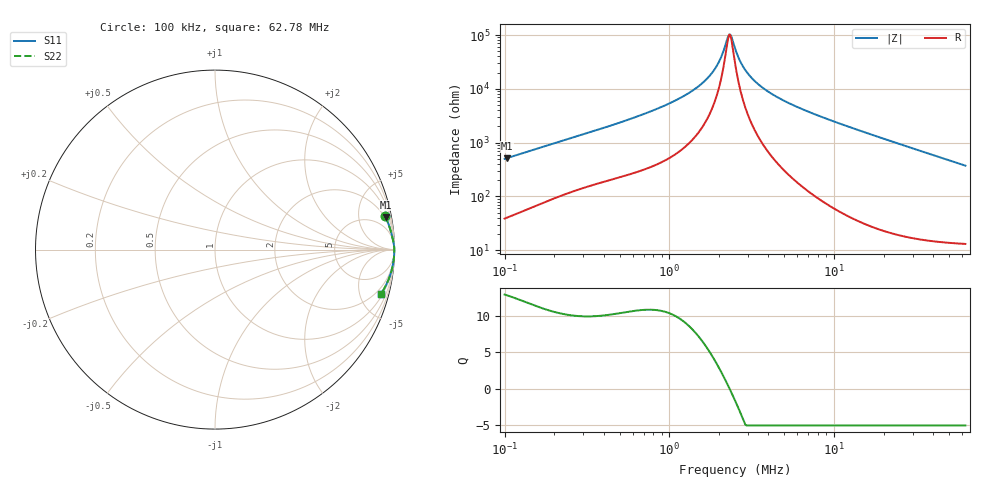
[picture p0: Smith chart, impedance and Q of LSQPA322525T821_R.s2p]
! LSQPA322525T821_R  S-PARAMETER MODEL  ( General Type )
! Model Generated by TAIYO YUDEN Corporation (http://www.ty-top.com)
! Version 1.0
! TAIYO YUDEN Control No. 111018NG25SB-FKC
! Copyright(c) 2011 TAIYO YUDEN CO.,LTD. All Rights Reserved.
! Product Description (link to TY-COMPAS)
! https://ds.yuden.co.jp/TYCOMPAS/or/detail?pn=LSQPA322525T821KR&u=M
! Products Name : Inductors
! Characteristics :
!  Inductance : 820 uH , SRF(min) : 1.8 MHz , DC Resistance(max) : 15.6 Ohm
!  Rated Current : Saturation :110 mA , Temp Rise : 110 mA (40 degC)
!  Case Size : 3.2 x 2.5 / 0.126 x 0.098 [mm/inch] , Thickness : 2.5 / 0.098 [mm/inch]
!  (Conditions: Temperature = 25 degC , DC Bias Current/Voltage = 0A / 0V)
! External Node Assignments :
!  1  o---GGG---o  2
! GND o---------o GND
! Frequency Range : 0.1MHz  -  62.782943MHz  [ 402 STEP ]
# MHz S RI R 50
! Freq[MHz].  S11 Real  S11 Imag  S21 Real  S21 Imag  S12 Real  S12 Imag  S22 Real  S22 Imag
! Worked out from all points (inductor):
!   401 points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, 100 kHz to 62.78 MHz, reference 50 ohm
!   read as one part in series: L = 782 uH near 103.3 kHz
!   highest Q = 12.8 at 103.3 kHz (marker M1), where L = 790 uH
!   self-resonance near 2.312 MHz
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0.1  0.9479 0.1867  0.0521 -0.1867  0.0521 -0.1867  0.9479 0.1867
0.103274  0.9504 0.1815  0.0496 -0.1815  0.0496 -0.1815  0.9504 0.1815
0.294197  0.9879 0.0699  0.0121 -0.0699  0.0121 -0.0699  0.9879 0.0699
0.551351  0.9949 0.0378  0.00507 -0.0378  0.00507 -0.0378  0.9949 0.0378
0.86552  0.9974 0.0225  0.00262 -0.0225  0.00262 -0.0225  0.9974 0.0225
1.273936  0.9984 0.0126  0.00158 -0.0126  0.00158 -0.0126  0.9984 0.0126
1.675158  0.9988 0.0066  0.00119 -0.0066  0.00119 -0.0066  0.9988 0.0066
1.815636  0.9989 0.00494  0.00112 -0.00494  0.00112 -0.00494  0.9989 0.00494
1.967894  0.9989 0.00332  0.00106 -0.00332  0.00106 -0.00332  0.9989 0.00332
2.098844  0.999 0.00203  0.00102 -0.00203  0.00102 -0.00203  0.999 0.00203
2.238508  0.999 0.000752  0.000983 -0.000752  0.000983 -0.000752  0.999 0.000752
2.311787  0.999 0.000113  0.000969 -0.000113  0.000969 -0.000113  0.999 0.000113
2.387465  0.999 -0.000526  0.000957 0.000526  0.000957 0.000526  0.999 -0.000526
2.546334  0.9991 -0.00181  0.000938 0.00181  0.000938 0.00181  0.9991 -0.00181
2.715775  0.9991 -0.0031  0.000925 0.0031  0.000925 0.0031  0.9991 -0.0031
2.896492  0.9991 -0.0044  0.000919 0.0044  0.000919 0.0044  0.9991 -0.0044
3.190362  0.9991 -0.00639  0.00092 0.00639  0.00092 0.00639  0.9991 -0.00639
3.571101  0.9991 -0.00879  0.00094 0.00879  0.00094 0.00879  0.9991 -0.00879
4.77205  0.9989 -0.0156  0.00109 0.0156  0.00109 0.0156  0.9989 -0.0156
7.371558  0.9983 -0.0284  0.00169 0.0284  0.00169 0.0284  0.9983 -0.0284
21.68692  0.9899 -0.0907  0.0101 0.0907  0.0101 0.0907  0.9899 -0.0907
62.78294  0.9253 -0.246  0.0747 0.246  0.0747 0.246  0.9253 -0.246
